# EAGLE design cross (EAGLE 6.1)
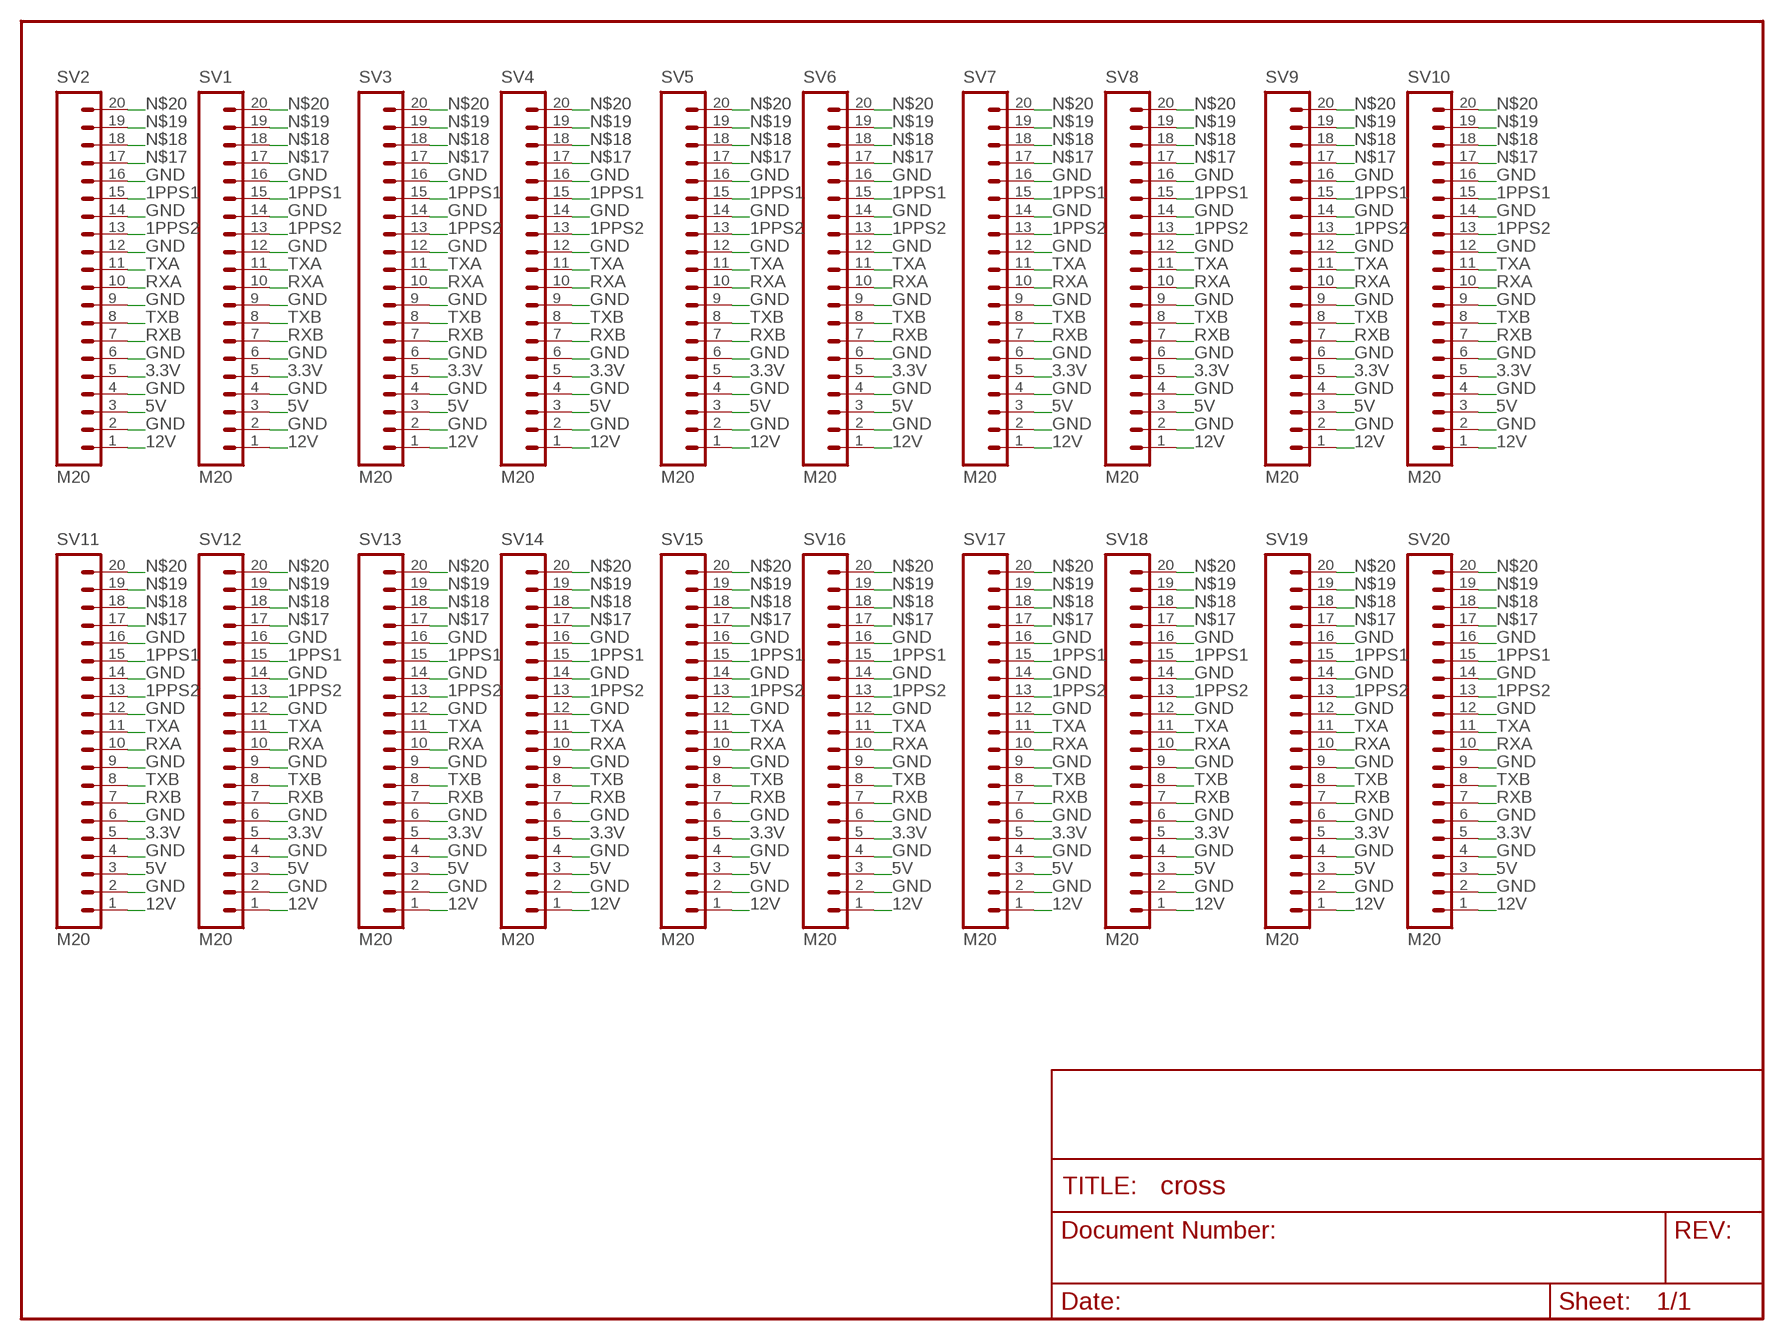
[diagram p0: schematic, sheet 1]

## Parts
SV1  M20  [1X20]
SV2  M20  [1X20]
SV3  M20  [1X20]
SV4  M20  [1X20]
SV5  M20  [1X20]
SV6  M20  [1X20]
SV7  M20  [1X20]
SV8  M20  [1X20]
SV9  M20  [1X20]
SV10  M20  [1X20]
SV11  M20  [1X20]
SV12  M20  [1X20]
SV13  M20  [1X20]
SV14  M20  [1X20]
SV15  M20  [1X20]
SV16  M20  [1X20]
SV17  M20  [1X20]
SV18  M20  [1X20]
SV19  M20  [1X20]
SV20  M20  [1X20]

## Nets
1PPS1: SV1.15 SV2.15 SV3.15 SV4.15 SV5.15 SV6.15 SV7.15 SV8.15 SV9.15 SV10.15 SV11.15 SV12.15 SV13.15 SV14.15 SV15.15 SV16.15 SV17.15 SV18.15 SV19.15 SV20.15
1PPS2: SV1.13 SV2.13 SV3.13 SV4.13 SV5.13 SV6.13 SV7.13 SV8.13 SV9.13 SV10.13 SV11.13 SV12.13 SV13.13 SV14.13 SV15.13 SV16.13 SV17.13 SV18.13 SV19.13 SV20.13
3.3V: SV1.5 SV2.5 SV3.5 SV4.5 SV5.5 SV6.5 SV7.5 SV8.5 SV9.5 SV10.5 SV11.5 SV12.5 SV13.5 SV14.5 SV15.5 SV16.5 SV17.5 SV18.5 SV19.5 SV20.5
5V: SV1.3 SV2.3 SV3.3 SV4.3 SV5.3 SV6.3 SV7.3 SV8.3 SV9.3 SV10.3 SV11.3 SV12.3 SV13.3 SV14.3 SV15.3 SV16.3 SV17.3 SV18.3 SV19.3 SV20.3
12V: SV1.1 SV2.1 SV3.1 SV4.1 SV5.1 SV6.1 SV7.1 SV8.1 SV9.1 SV10.1 SV11.1 SV12.1 SV13.1 SV14.1 SV15.1 SV16.1 SV17.1 SV18.1 SV19.1 SV20.1
GND: SV1.2 SV1.4 SV1.6 SV1.9 SV1.12 SV1.14 SV1.16 SV2.2 SV2.4 SV2.6 SV2.9 SV2.12 SV2.14 SV2.16 SV3.2 SV3.4 SV3.6 SV3.9 SV3.12 SV3.14 SV3.16 SV4.2 SV4.4 SV4.6 SV4.9 SV4.12 SV4.14 SV4.16 SV5.2 SV5.4 SV5.6 SV5.9 SV5.12 SV5.14 SV5.16 SV6.2 SV6.4 SV6.6 SV6.9 SV6.12 SV6.14 SV6.16 SV7.2 SV7.4 SV7.6 SV7.9 SV7.12 SV7.14 SV7.16 SV8.2 SV8.4 SV8.6 SV8.9 SV8.12 SV8.14 SV8.16 SV9.2 SV9.4 SV9.6 SV9.9 SV9.12 SV9.14 SV9.16 SV10.2 SV10.4 SV10.6 SV10.9 SV10.12 SV10.14 SV10.16 SV11.2 SV11.4 SV11.6 SV11.9 SV11.12 SV11.14 SV11.16 SV12.2 SV12.4 SV12.6 SV12.9 SV12.12 SV12.14 SV12.16 SV13.2 SV13.4 SV13.6 SV13.9 SV13.12 SV13.14 SV13.16 SV14.2 SV14.4 SV14.6 SV14.9 SV14.12 SV14.14 SV14.16 SV15.2 SV15.4 SV15.6 SV15.9 SV15.12 SV15.14 SV15.16 SV16.2 SV16.4 SV16.6 SV16.9 SV16.12 SV16.14 SV16.16 SV17.2 SV17.4 SV17.6 SV17.9 SV17.12 SV17.14 SV17.16 SV18.2 SV18.4 SV18.6 SV18.9 SV18.12 SV18.14 SV18.16 SV19.2 SV19.4 SV19.6 SV19.9 SV19.12 SV19.14 SV19.16 SV20.2 SV20.4 SV20.6 SV20.9 SV20.12 SV20.14 SV20.16
N$17: SV1.17 SV2.17 SV3.17 SV4.17 SV5.17 SV6.17 SV7.17 SV8.17 SV9.17 SV10.17 SV11.17 SV12.17 SV13.17 SV14.17 SV15.17 SV16.17 SV17.17 SV18.17 SV19.17 SV20.17
N$18: SV1.18 SV2.18 SV3.18 SV4.18 SV5.18 SV6.18 SV7.18 SV8.18 SV9.18 SV10.18 SV11.18 SV12.18 SV13.18 SV14.18 SV15.18 SV16.18 SV17.18 SV18.18 SV19.18 SV20.18
N$19: SV1.19 SV2.19 SV3.19 SV4.19 SV5.19 SV6.19 SV7.19 SV8.19 SV9.19 SV10.19 SV11.19 SV12.19 SV13.19 SV14.19 SV15.19 SV16.19 SV17.19 SV18.19 SV19.19 SV20.19
N$20: SV1.20 SV2.20 SV3.20 SV4.20 SV5.20 SV6.20 SV7.20 SV8.20 SV9.20 SV10.20 SV11.20 SV12.20 SV13.20 SV14.20 SV15.20 SV16.20 SV17.20 SV18.20 SV19.20 SV20.20
RXA: SV1.10 SV2.10 SV3.10 SV4.10 SV5.10 SV6.10 SV7.10 SV8.10 SV9.10 SV10.10 SV11.10 SV12.10 SV13.10 SV14.10 SV15.10 SV16.10 SV17.10 SV18.10 SV19.10 SV20.10
RXB: SV1.7 SV2.7 SV3.7 SV4.7 SV5.7 SV6.7 SV7.7 SV8.7 SV9.7 SV10.7 SV11.7 SV12.7 SV13.7 SV14.7 SV15.7 SV16.7 SV17.7 SV18.7 SV19.7 SV20.7
TXA: SV1.11 SV2.11 SV3.11 SV4.11 SV5.11 SV6.11 SV7.11 SV8.11 SV9.11 SV10.11 SV11.11 SV12.11 SV13.11 SV14.11 SV15.11 SV16.11 SV17.11 SV18.11 SV19.11 SV20.11
TXB: SV1.8 SV2.8 SV3.8 SV4.8 SV5.8 SV6.8 SV7.8 SV8.8 SV9.8 SV10.8 SV11.8 SV12.8 SV13.8 SV14.8 SV15.8 SV16.8 SV17.8 SV18.8 SV19.8 SV20.8

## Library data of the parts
SV1-SV20 = SparkFun:M20: This is just like the LOCK variant in that the holes are staggared by 5 mil, but except for the last two holes. They are not altered from the "standard" footprint layout. This is used for a special purpose on the layout of our Graphic LCD Backpack. Make sure you want to use this device before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

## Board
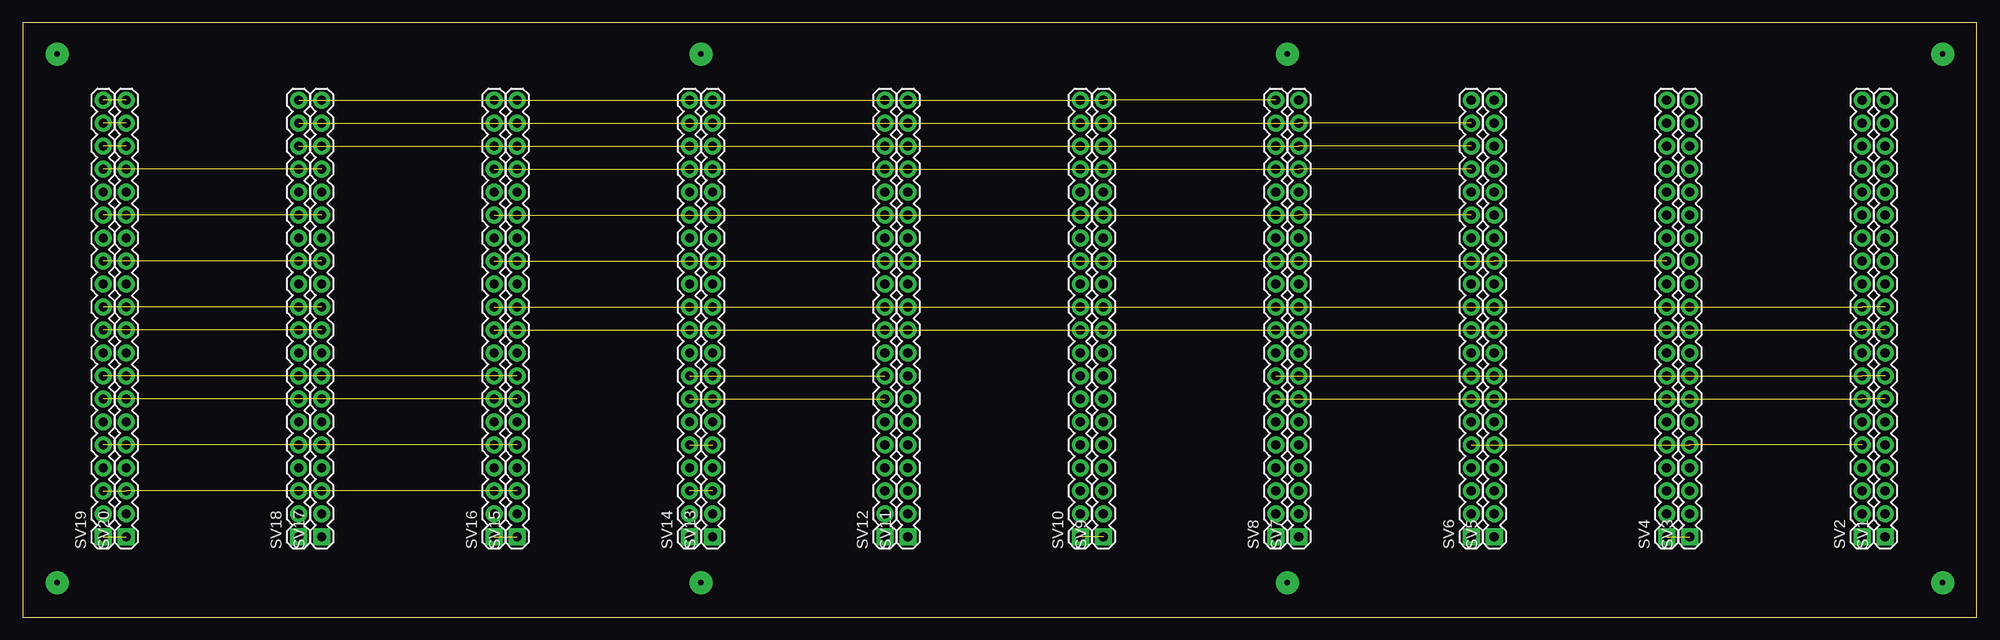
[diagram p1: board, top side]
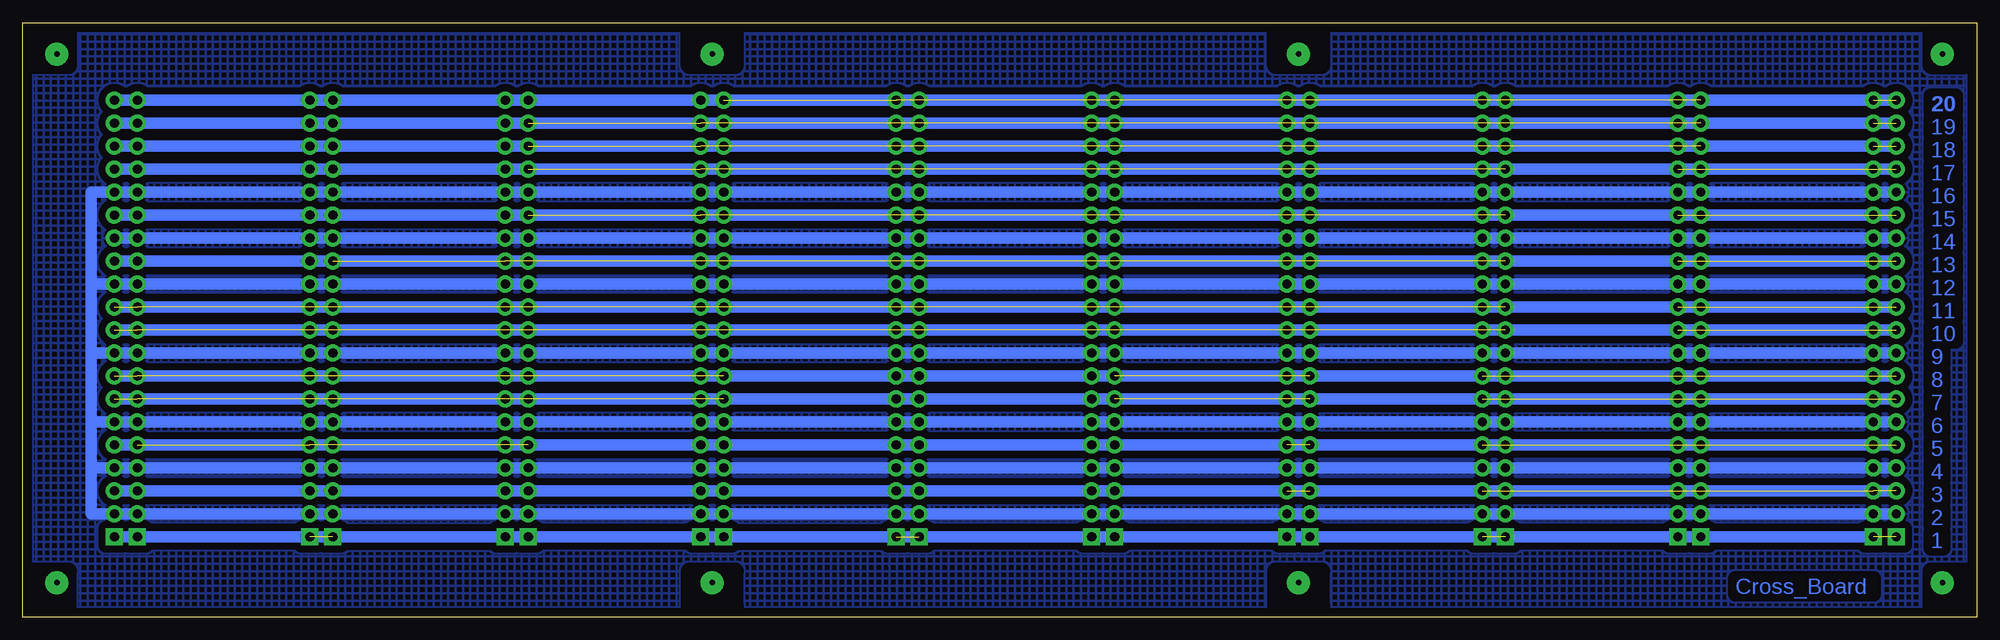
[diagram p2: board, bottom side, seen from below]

Size 215.88 x 65.71 mm. Coordinates in mm from the lower left corner, seen from the top.
Outline: 0,0 215.88,0 215.88,65.71 0,65.71 0,0
Copper layers (1*16): Top 0.035mm / dielectric 1.5mm / Bottom 0.035mm
Design rules: minimum track width 10mil, minimum drill 24mil, track to track 8mil, track to pad 8mil, pad to pad 8mil, via to via 8mil, smd to smd 8mil, copper to edge 40mil, drill to drill 8mil, minimum pad ring 10mil, minimum via ring 8mil, stop-mask expansion 4mil, vias tented up to drill 0mil, thermal gap 10mil
bRestrict: 32 lines

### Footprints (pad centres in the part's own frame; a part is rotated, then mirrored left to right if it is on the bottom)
1X20 = drill 1.016 pad 1.88 square: 1 0,0 | drill 1.016 pad 1.88: 2 2.54,0; 3 5.08,0; 4 7.62,0; 5 10.16,0; 6 12.7,0; 7 15.24,0; 8 17.78,0; 9 20.32,0; 10 22.86,0; 11 25.4,0; 12 27.94,0; 13 30.48,0; 14 33.02,0; 15 35.56,0; 16 38.1,0; 17 40.64,0; 18 43.18,0; 19 45.72,0; 20 48.26,0

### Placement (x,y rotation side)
SV1  205.74,8.89 90 top
SV2  203.2,8.89 90 top
SV3  184.15,8.89 90 top
SV4  181.61,8.89 90 top
SV5  162.56,8.89 90 top
SV6  160.02,8.89 90 top
SV7  140.97,8.89 90 top
SV8  138.43,8.89 90 top
SV9  119.38,8.89 90 top
SV10  116.84,8.89 90 top
SV11  97.79,8.89 90 top
SV12  95.25,8.89 90 top
SV13  76.2,8.89 90 top
SV14  73.66,8.89 90 top
SV15  54.61,8.89 90 top
SV16  52.07,8.89 90 top
SV17  33.02,8.89 90 top
SV18  30.48,8.89 90 top
SV19  8.89,8.89 90 top
SV20  11.43,8.89 90 top

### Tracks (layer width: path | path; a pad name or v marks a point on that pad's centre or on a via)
1PPS1  (13 unrouted)
  Bottom 0.254: SV2.15 SV4.15
  Bottom 1.27: SV1.15 SV2.15 SV3.15 SV4.15 SV5.15 SV6.15 SV19.15
1PPS2  (15 unrouted)
  Bottom 1.27: SV1.13 SV2.13 SV3.13 SV4.13 SV19.13
3.3V  (10 unrouted)
  Bottom 1.27: SV19.5 SV13.5 SV12.5 SV11.5 SV10.5 SV9.5 SV8.5 SV7.5 SV2.5 SV1.5
5V  (6 unrouted)
  Bottom 1.27: SV1.3 SV2.3 SV3.3 SV4.3 SV5.3 SV6.3 SV7.3 SV8.3 SV9.3 SV10.3 SV11.3 SV12.3 SV14.3 SV19.3
12V  (4 unrouted)
  Bottom 1.27: SV1.1 SV2.1 SV4.1 SV5.1 SV6.1 SV7.1 SV8.1 SV10.1 SV11.1 SV12.1 SV13.1 SV14.1 SV15.1 SV17.1 SV18.1 SV20.1
GND
  Bottom 1.27: SV3.4 SV2.4 SV1.4 208.28,16.51 | SV3.4 SV4.4 | SV3.4 SV5.4 SV7.4 SV8.4 SV9.4 | SV9.2 SV8.2 SV6.2 SV5.2 SV4.2 SV3.2 208.28,11.43 208.28,16.51 | SV10.2 SV9.2 | SV9.2 SV11.2 SV12.2 SV19.2 | SV9.4 SV10.4 | SV9.4 SV11.4 SV12.4 SV19.4 | SV19.14 SV2.14 SV1.14 | SV19.12 SV1.12 208.28,36.83 | SV19.9 SV12.9 SV11.9 SV10.9 SV1.9 208.28,29.21 | SV19.6 SV12.6 SV11.6 SV10.6 SV9.6 SV7.6 | SV8.6 SV7.6 | SV7.6 SV2.6 SV1.6 208.28,21.59 | SV19.16 SV20.16 SV2.16 SV1.16 208.28,46.99 208.28,36.83 | 208.28,16.51 208.28,21.59 | 208.28,21.59 208.28,29.21 | 208.28,29.21 208.28,36.83
  pour Bottom (isolate 0.813, hatched): 0,66.04 0,0 217.17,0 215.9,66.04
N$2  (via drill 0.6 pad 2.54)
  other vias: 3.81,62.23
N$3  (via drill 0.6 pad 2.54)
  other vias: 74.93,62.23
N$4  (via drill 0.6 pad 2.54)
  other vias: 139.7,62.23
N$6  (via drill 0.6 pad 2.54)
  other vias: 212.09,62.23
N$7  (via drill 0.6 pad 2.54)
  other vias: 3.81,3.81
N$8  (via drill 0.6 pad 2.54)
  other vias: 74.93,3.81
N$9  (via drill 0.6 pad 2.54)
  other vias: 139.7,3.81
N$10  (via drill 0.6 pad 2.54)
  other vias: 212.09,3.81
N$17  (13 unrouted)
  Bottom 1.27: SV19.17 SV6.17 SV5.17 SV4.17 SV3.17 SV2.17 SV1.17
N$18  (13 unrouted)
  Bottom 0.254: SV3.18 SV5.18
  Bottom 1.27: SV1.18 SV2.18 SV3.18 SV4.18 SV5.18 SV6.18 SV19.18
N$19  (13 unrouted)
  Bottom 1.27: SV19.19 SV6.19 SV5.19 163.83,54.61 SV4.19 SV3.19 SV2.19 SV1.19
N$20  (11 unrouted)
  Bottom 1.27: SV1.20 SV2.20 SV3.20 SV4.20 SV5.20 SV6.20 SV7.20 SV8.20 SV19.20
RXA  (18 unrouted)
  Bottom 1.27: SV1.10 SV19.10
RXB  (14 unrouted)
  Bottom 1.27: SV19.7 SV12.7 SV11.7 SV10.7 SV9.7 SV1.7
TXA  (18 unrouted)
  Bottom 1.27: SV19.11 SV1.11
TXB  (14 unrouted)
  Bottom 1.27: SV19.8 SV12.8 SV11.8 SV10.8 SV9.8 SV1.8

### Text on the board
Bottom: 20 | 19 | 18 | 17 | 16 | 15 | 14 | 13 | 12 | 11 | 10 | 9 | 8 | 7 | 6 | 5 | 4 | 3 | 2 | 1 | Cross_Board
